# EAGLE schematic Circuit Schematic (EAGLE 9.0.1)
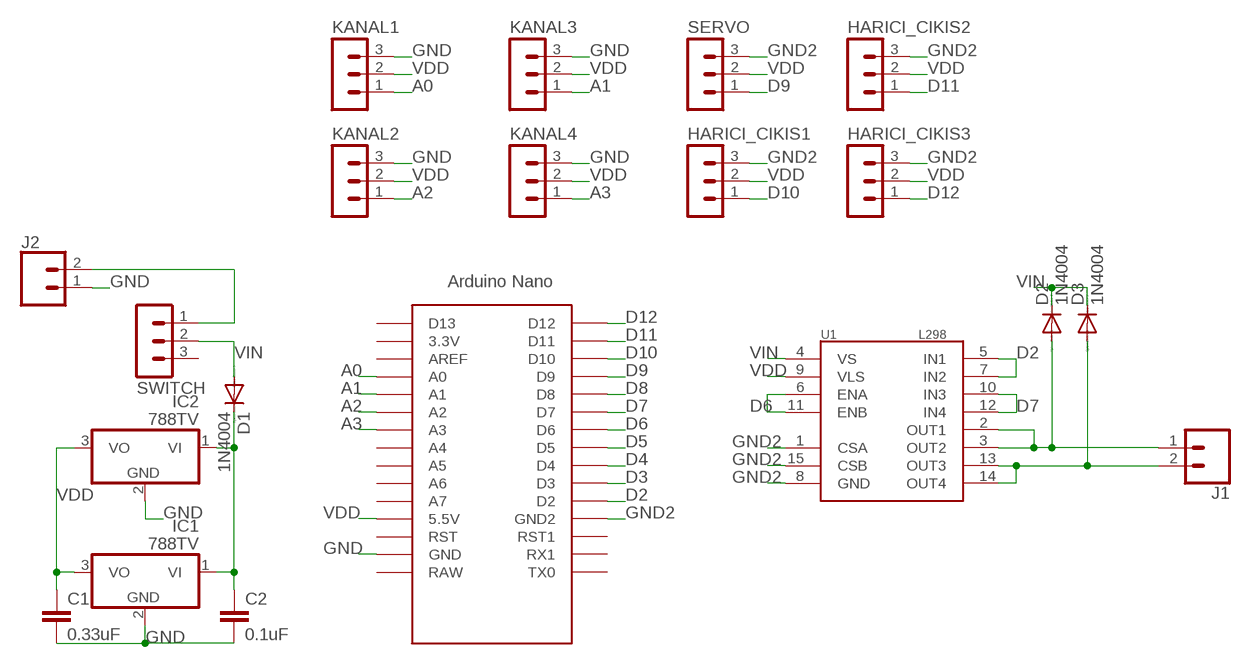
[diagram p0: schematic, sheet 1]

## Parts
C1  0.33uF  C2.5/2  [C2.5-2]
C2  0.1uF  C2.5/2  [C2.5-2]
D1  1N4004  [DO41-10]
D2  1N4004  [DO41-10]
D3  1N4004  [DO41-10]
HARICI_CIKIS1  MA03-1  [MA03-1]
HARICI_CIKIS2  MA03-1  [MA03-1]
HARICI_CIKIS3  MA03-1  [MA03-1]
IC1  788TV  [TO220V]
IC2  788TV  [TO220V]
J1  CONN_025MM  [SCREWTERMINAL-5MM-2]
J2  CONN_025MM  [SCREWTERMINAL-5MM-2]
KANAL1  MA03-1  [MA03-1]
KANAL2  MA03-1  [MA03-1]
KANAL3  MA03-1  [MA03-1]
KANAL4  MA03-1  [MA03-1]
SERVO  MA03-1  [MA03-1]
SWITCH  MA03-1  [MA03-1]
U1  L298  [MULTIWATT15]
U$1  NANO  [NANO]

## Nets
A0: KANAL1.1 U$1.A0
A1: KANAL3.1 U$1.A1
A2: KANAL2.1 U$1.A2
A3: KANAL4.1 U$1.A3
D2: U1.5(IN1) U1.7(IN2) U$1.D2
D3: U$1.D3
D4: U$1.D4
D5: U$1.D5
D6: U1.6(ENA) U1.11(ENB) U$1.D6
D7: U1.10(IN3) U1.12(IN4) U$1.D7
D8: U$1.D8
D9: SERVO.1 U$1.D9
D10: HARICI_CIKIS1.1 U$1.D10
D11: HARICI_CIKIS2.1 U$1.D11
D12: HARICI_CIKIS3.1 U$1.D12
DVıN: C2.1 D1.C IC1.1(VI) IC2.1(VI)
GND: C1.2 C2.2 IC1.2(GND) IC2.2(GND) J2.1 KANAL1.3 KANAL2.3 KANAL3.3 KANAL4.3 U$1.GND
GND2: HARICI_CIKIS1.3 HARICI_CIKIS2.3 HARICI_CIKIS3.3 SERVO.3 U1.1(CSA) U1.8(GND) U1.15(CSB) U$1.GND1(GND2)
N$1: D2.A J1.1 U1.2(OUT1) U1.3(OUT2)
N$3: J2.2 SWITCH.1
N$4: D3.A J1.2 U1.13(OUT3) U1.14(OUT4)
VDD: C1.1 HARICI_CIKIS1.2 HARICI_CIKIS2.2 HARICI_CIKIS3.2 IC1.3(VO) IC2.3(VO) KANAL1.2 KANAL2.2 KANAL3.2 KANAL4.2 SERVO.2 U1.9(VLS) U$1.5V(5.5V)
VIN: D1.A D2.C D3.C SWITCH.2 U1.4(VS)
Unconnected: SWITCH.3 U$1.3.3V U$1.A4 U$1.A5 U$1.A6 U$1.A7 U$1.AREF U$1.D13 U$1.ICSP1 U$1.ICSP2 U$1.ICSP3 U$1.ICSP4 U$1.ICSP5 U$1.ICSP6 U$1.RAW U$1.RST U$1.RST1 U$1.RX1 U$1.TX0

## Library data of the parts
C1 C2 = capacitor-wima:C: CAPACITOR
D1-D3 = diode:1N4004: DIODE
HARICI_CIKIS1-HARICI_CIKIS3 KANAL1-KANAL4 SERVO SWITCH = con-lstb:MA03-1: PIN HEADER; OC_FARNELL: unknown; OC_NEWARK: unknown
IC1 IC2 = linear:78*: Positive VOLTAGE REGULATOR Source: http://cache.national.com/ds/LM/LM78L05.pdf http://www.fairchildsemi.com/ds/LM/LM7805.pdf
J1 J2 = SparkFun-Connectors:CONN_02: Multi connection point. Often used as Generic Header-pin footprint for 0.1 inch spaced/style header connections; SF_SKU: PRT-08432
U1 = SparkFun-IC-Special-Function:L298: L298 Dual Full Bridge Driver
U$1 = Arduino:NANO: Arduino Nano

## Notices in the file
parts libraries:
SparkFun-IC-Special-Function: Licensing: Creative Commons ShareAlike 4.0 International - https://creativecommons.org/licenses/by-sa/4.0
